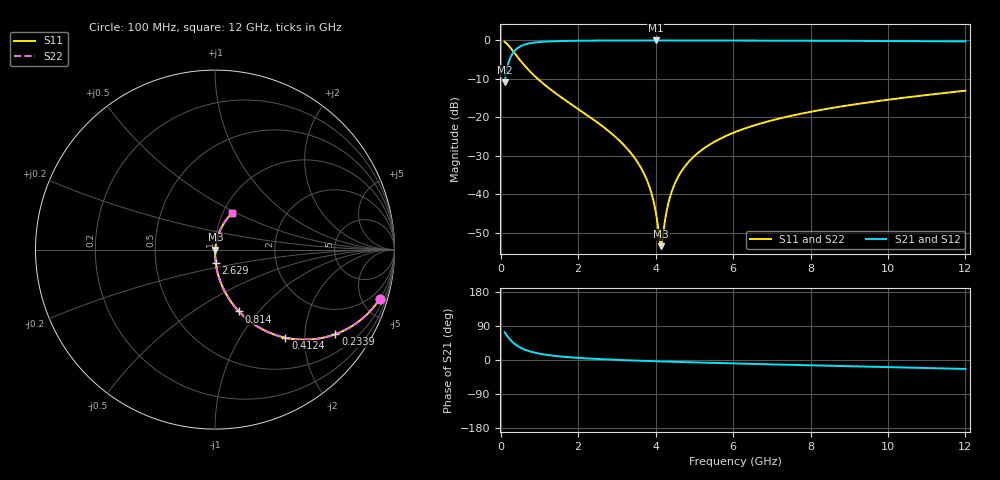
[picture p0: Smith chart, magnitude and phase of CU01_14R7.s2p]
! S-parameter model data by Modelithics Inc. support@modelithics.com 813-866-6335 Tampa FL USA
! S-Parameter data specifications:
! Substrate: 20-mil Rogers, substrate thickness, H=0.508mm, Dielectric constant, Er=3.75
! PCB Mounting Pad Footprint: Pad width, PadW=0.35mm , Pad length, PadL=0.30mm , Pad gap, PadG (edge-to-edge)=0.25mm , Reference planes=0.85mm apart
! Created Tue May  8 14:01:25 2018
# hz S ma R 50
! 2 Port Network Data from SP1.SP block
! freq  magS11  angS11  magS21  angS21  magS12  angS12  magS22  angS22
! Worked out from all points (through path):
!   801 points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, 100 MHz to 12 GHz, reference 50 ohm
!   highest |S21| = -0.02 dB at 3.997 GHz (marker M1); lowest = -10.9 dB at 100 MHz (marker M2)
!   group delay of S21, straight-line fit = 11 ps
!   lowest |S11| = -53.5 dB at 4.146 GHz (marker M3), VSWR 1.00, Z = 50.2 + j0.00955 ohm
!   |S11| at or under -10 dB: 955.2 MHz to end of sweep
!   |S22| runs from -53.5 to -0.4 dB; largest |S21 - S12| = 0
!   S11 on the Smith chart (normalised r, x): 100 MHz: 0.99, -6.69; 233.9 MHz: 0.99, -2.85; 412.4 MHz: 0.99, -1.61; 814 MHz: 0.99, -0.79; 2.629 GHz: 1.00, -0.15; 12 GHz: 1.10, +0.47
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1e8  0.9584 -16.6  0.2849 73.3  0.2849 73.3  0.9584 -16.6
2.33875e8  0.82 -35.1  0.5717 54.9  0.5717 54.9  0.82 -35.1
4.12375e8  0.6281 -51.4  0.7773 38.5  0.7773 38.5  0.6281 -51.4
5.90875e8  0.4869 -61.3  0.8725 28.6  0.8725 28.6  0.4869 -61.3
8.14e8  0.3691 -68.9  0.9283 20.9  0.9283 20.9  0.3691 -68.9
1.275125e9  0.2322 -77.4  0.9713 12.3  0.9713 12.3  0.2322 -77.4
2.09325e9  0.1189 -84.3  0.9913 4.9  0.9913 4.9  0.1189 -84.3
2.62875e9  0.07634 -86.7  0.9953 2.0  0.9953 2.0  0.07634 -86.7
3.179125e9  0.04357 -87.9  0.9971 -0.4  0.9971 -0.4  0.04357 -87.9
3.565875e9  0.02454 -87.2  0.9977 -1.8  0.9977 -1.8  0.02454 -87.2
3.833625e9  0.01274 -83.6  0.9978 -2.7  0.9978 -2.7  0.01274 -83.6
3.99725e9  0.006101 -73.6  0.9979 -3.3  0.9979 -3.3  0.006101 -73.6
4.071625e9  0.003427 -56.3  0.9979 -3.5  0.9979 -3.5  0.003427 -56.3
4.146e9  0.002103 2.6  0.9978 -3.8  0.9978 -3.8  0.002103 2.6
4.190625e9  0.002889 39.5  0.9978 -3.9  0.9978 -3.9  0.002889 39.5
4.384e9  0.009619 72.6  0.9977 -4.5  0.9977 -4.5  0.009619 72.6
4.696375e9  0.02084 78.5  0.9975 -5.4  0.9975 -5.4  0.02084 78.5
5.231875e9  0.03886 79.6  0.9969 -6.9  0.9969 -6.9  0.03886 79.6
6.05e9  0.06406 78.7  0.9954 -9.1  0.9954 -9.1  0.06406 78.7
8.04325e9  0.1188 74.5  0.9899 -14.1  0.9899 -14.1  0.1188 74.5
1.002162e10  0.1695 70.0  0.9819 -18.8  0.9819 -18.8  0.1695 70.0
1.2e10  0.2217 65.2  0.9702 -23.6  0.9702 -23.6  0.2217 65.2
